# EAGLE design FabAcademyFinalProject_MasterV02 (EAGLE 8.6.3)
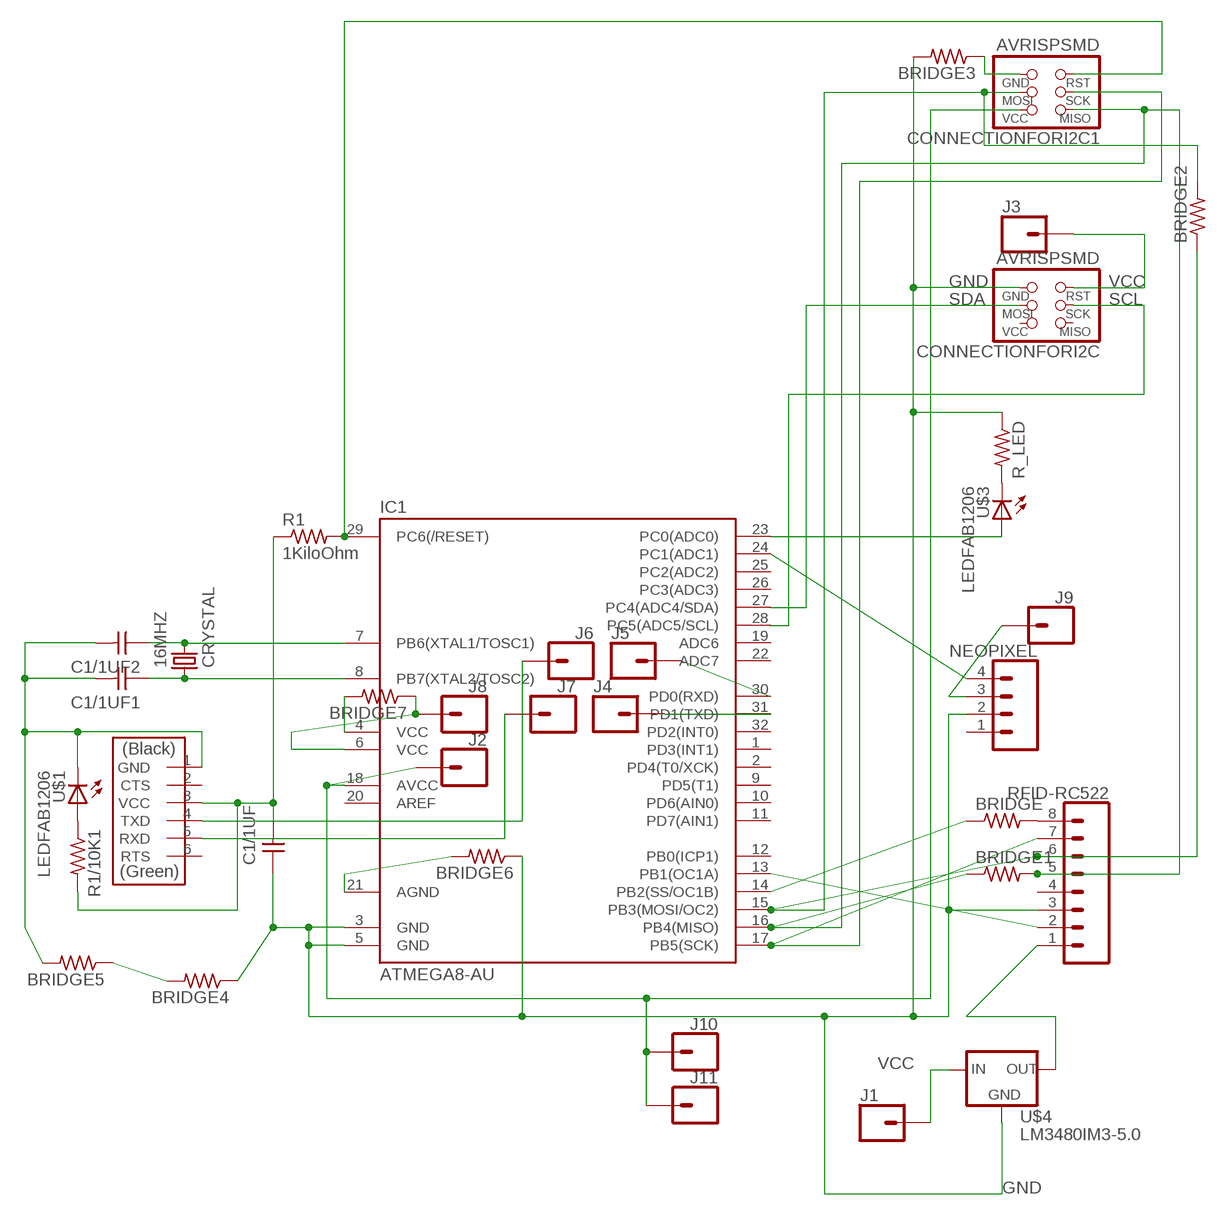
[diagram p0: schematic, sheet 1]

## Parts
16MHZ  CRYSTAL  [2-SMD-5X3MM]
BRIDGE  RES-US1206FAB  [R1206FAB]
BRIDGE1  RES-US1206FAB  [R1206FAB]
BRIDGE2  RES-US1206FAB  [R1206FAB]
BRIDGE3  RES-US1206FAB  [R1206FAB]
BRIDGE4  RES-US1206FAB  [R1206FAB]
BRIDGE5  RES-US1206FAB  [R1206FAB]
BRIDGE6  RES-US1206FAB  [R1206FAB]
BRIDGE7  RES-US1206FAB  [R1206FAB]
C1/1UF  CAP-UNPOLARIZEDFAB  [C1206FAB]
C1/1UF1  CAP-UNPOLARIZEDFAB  [C1206FAB]
C1/1UF2  CAP-UNPOLARIZEDFAB  [C1206FAB]
CONNECTIONFORI2C  AVRISPSMD  [2X03SMD]
CONNECTIONFORI2C1  AVRISPSMD  [2X03SMD]
IC1  ATMEGA8-AU  [TQFP32-08]
J1  CONN_01  [1X01]
J2  CONN_01  [1X01]
J3  CONN_01  [1X01]
J4  CONN_01  [1X01]
J5  CONN_01  [1X01]
J6  CONN_01  [1X01]
J7  CONN_01  [1X01]
J8  CONN_01  [1X01]
J9  CONN_01  [1X01]
J10  CONN_01  [1X01]
J11  CONN_01  [1X01]
NEOPIXEL  CONN_04  [1X04]
R1  1KiloOhm  RES-US1206FAB  [R1206FAB]
R1/10K1  RES-US1206FAB  [R1206FAB]
R_LED  RES-US1206FAB  [R1206FAB]
RFID-RC522  CONN_08"  [1X08]
U$1  LEDFAB1206  [LED1206FAB]
U$2  FTDI-SMD-HEADER  [1X06SMD]
U$3  LEDFAB1206  [LED1206FAB]
U$4  LM3480IM3-5.0  [SOT23]

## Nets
3.3V: RFID-RC522.1 U$4.1(OUT)
DI: IC1.24(PC1(ADC1)) NEOPIXEL.4
GND: BRIDGE3.2 BRIDGE4.1 BRIDGE5.2 BRIDGE6.1 C1/1UF1.2 C1/1UF2.2 C1/1UF.1 CONNECTIONFORI2C.6(GND) IC1.3(GND) IC1.5(GND) NEOPIXEL.2 R_LED.1 RFID-RC522.3 U$1.2(C) U$2.1(GND) U$4.3(GND)
N$1: IC1.13(PB1(OC1A)) RFID-RC522.2
N$2: CONNECTIONFORI2C1.3(SCK) IC1.17(PB5(SCK)) RFID-RC522.7
N$3: BRIDGE3.1 CONNECTIONFORI2C1.6(GND)
N$4: BRIDGE1.1 BRIDGE1.2 CONNECTIONFORI2C1.1(MISO) IC1.16(PB4(MISO)) RFID-RC522.5
N$5: BRIDGE.1 IC1.14(PB2(SS/OC1B))
N$6: 16MHZ.P$2 C1/1UF2.1 IC1.7(PB6(XTAL1/TOSC1))
N$7: 16MHZ.P$1 C1/1UF1.1 IC1.8(PB7(XTAL2/TOSC2))
N$8: J6.1 U$2.4(TXD)
N$9: R_LED.2 U$3.2(C)
N$10: IC1.23(PC0(ADC0)) U$3.1(A)
N$11: J7.1 U$2.5(RXD)
N$12: R1/10K1.1 U$1.1(A)
N$13: CONNECTIONFORI2C1.5(RST) IC1.29(PC6(/RESET)) R1.2
N$14: BRIDGE.2 RFID-RC522.8
N$15: BRIDGE2.1 BRIDGE2.2 CONNECTIONFORI2C1.4(MOSI) IC1.15(PB3(MOSI/OC2)) RFID-RC522.6
N$16: BRIDGE6.2 IC1.21(AGND)
N$17: BRIDGE4.2 BRIDGE5.1
N$18: IC1.30(PD0(RXD)) J5.1
N$19: IC1.31(PD1(TXD)) J4.1
N$20: BRIDGE7.2 IC1.4(VCC)
SCL: CONNECTIONFORI2C.3(SCK) IC1.28(PC5(ADC5/SCL))
SDA: CONNECTIONFORI2C.4(MOSI) IC1.27(PC4(ADC4/SDA))
VCC: BRIDGE7.1 C1/1UF.2 CONNECTIONFORI2C1.2(VCC) CONNECTIONFORI2C.5(RST) IC1.6(VCC) IC1.18(AVCC) J1.1 J2.1 J3.1 J8.1 J9.1 J10.1 J11.1 NEOPIXEL.3 R1.1 R1/10K1.2 U$2.3(VCC) U$4.2(IN)
Unconnected: CONNECTIONFORI2C.1(MISO) CONNECTIONFORI2C.2(VCC) IC1.1(PD3(INT1)) IC1.2(PD4(T0/XCK)) IC1.9(PD5(T1)) IC1.10(PD6(AIN0)) IC1.11(PD7(AIN1)) IC1.12(PB0(ICP1)) IC1.19(ADC6) IC1.20(AREF) IC1.22(ADC7) IC1.25(PC2(ADC2)) IC1.26(PC3(ADC3)) IC1.32(PD2(INT0)) NEOPIXEL.1 RFID-RC522.4 U$2.2(CTS) U$2.6(RTS)

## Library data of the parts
16MHZ = fab:CRYSTAL
BRIDGE BRIDGE1-BRIDGE7 R1 R1/10K1 R_LED = fab:RES-US: Resistor (US Symbol)
C1/1UF C1/1UF1 C1/1UF2 = fab:CAP-UNPOLARIZED
CONNECTIONFORI2C CONNECTIONFORI2C1 = fab:AVRISP
IC1 = atmega8:ATMEGA8
J1-J11 = SparkFun-Connectors:CONN_01: Single connection point. Often used as Generic Header-pin footprint for 0.1 inch spaced/style header connections
NEOPIXEL = SparkFun-Connectors:CONN_04: Multi connection point. Often used as Generic Header-pin footprint for 0.1 inch spaced/style header connections On any of the 0.1 inch spaced packages, you can populate with these: Break Away Headers - Straight (PRT-00116) Break Away Male Headers - Right Angle (PRT-00553) Female Headers (PRT-00115)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; PROD_ID: CONN-09696
RFID-RC522 = SparkFun-Connectors:CONN_08: Multi connection point. Often used as Generic Header-pin footprint for 0.1 inch spaced/style header connections On any of the 0.1 inch spaced packages, you can populate with these: Break Away Headers - Straight (PRT-00116) Break Away Male Headers - Right Angle (PRT-00553) Female Headers (PRT-00115)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; PROD_ID: CONN-08438
U$1 U$3 = fab:LED: LED
U$2 = fab:FTDI-SMD-HEADER
U$4 = national_gaui:LM3480

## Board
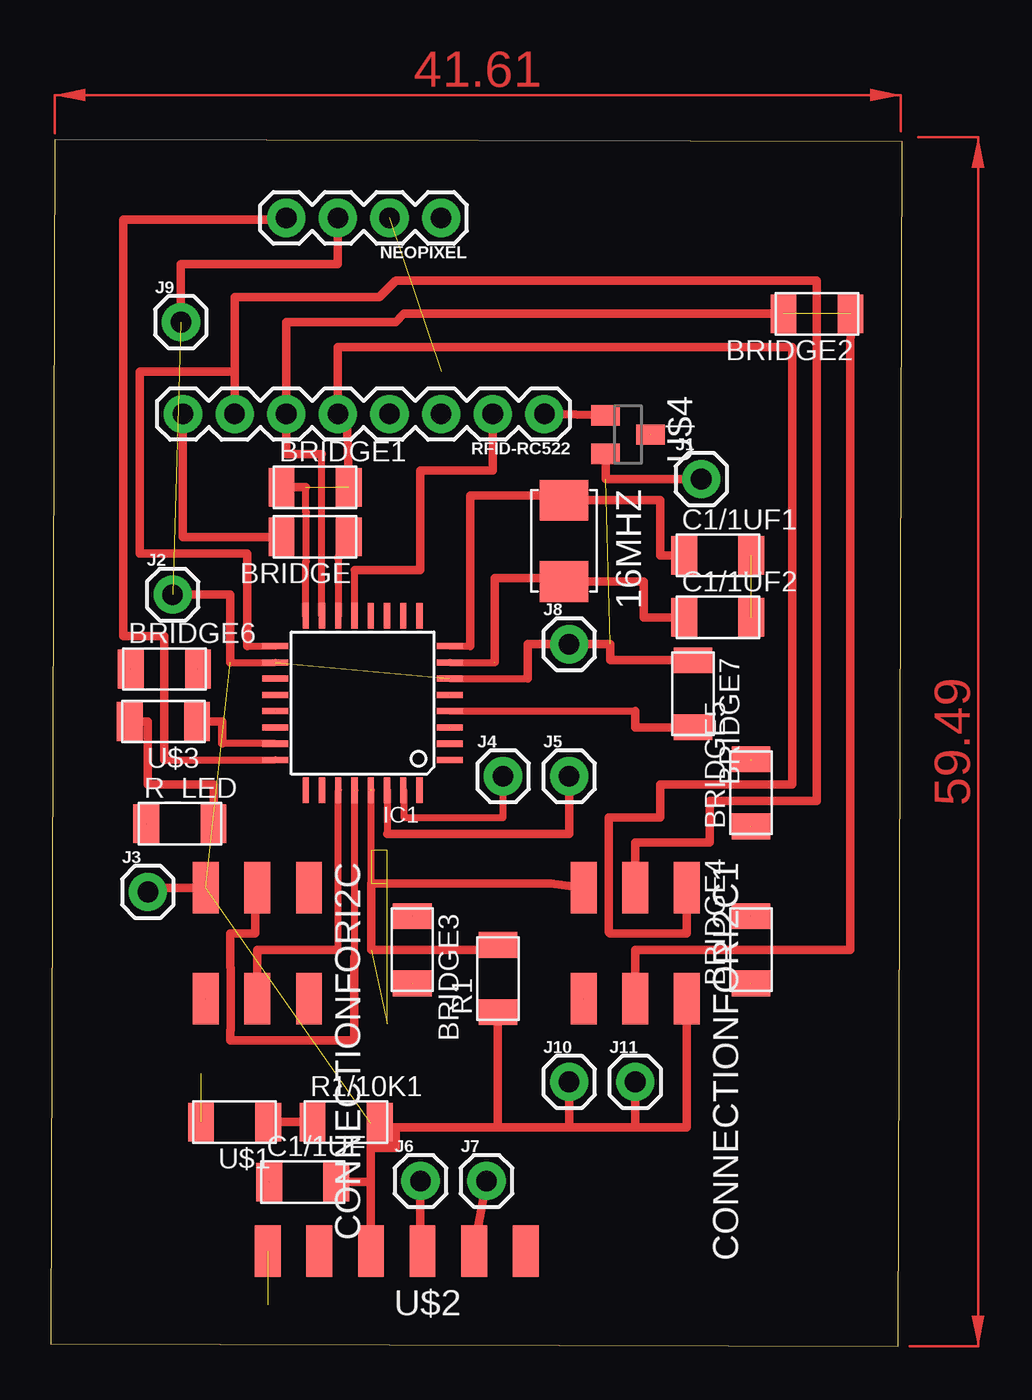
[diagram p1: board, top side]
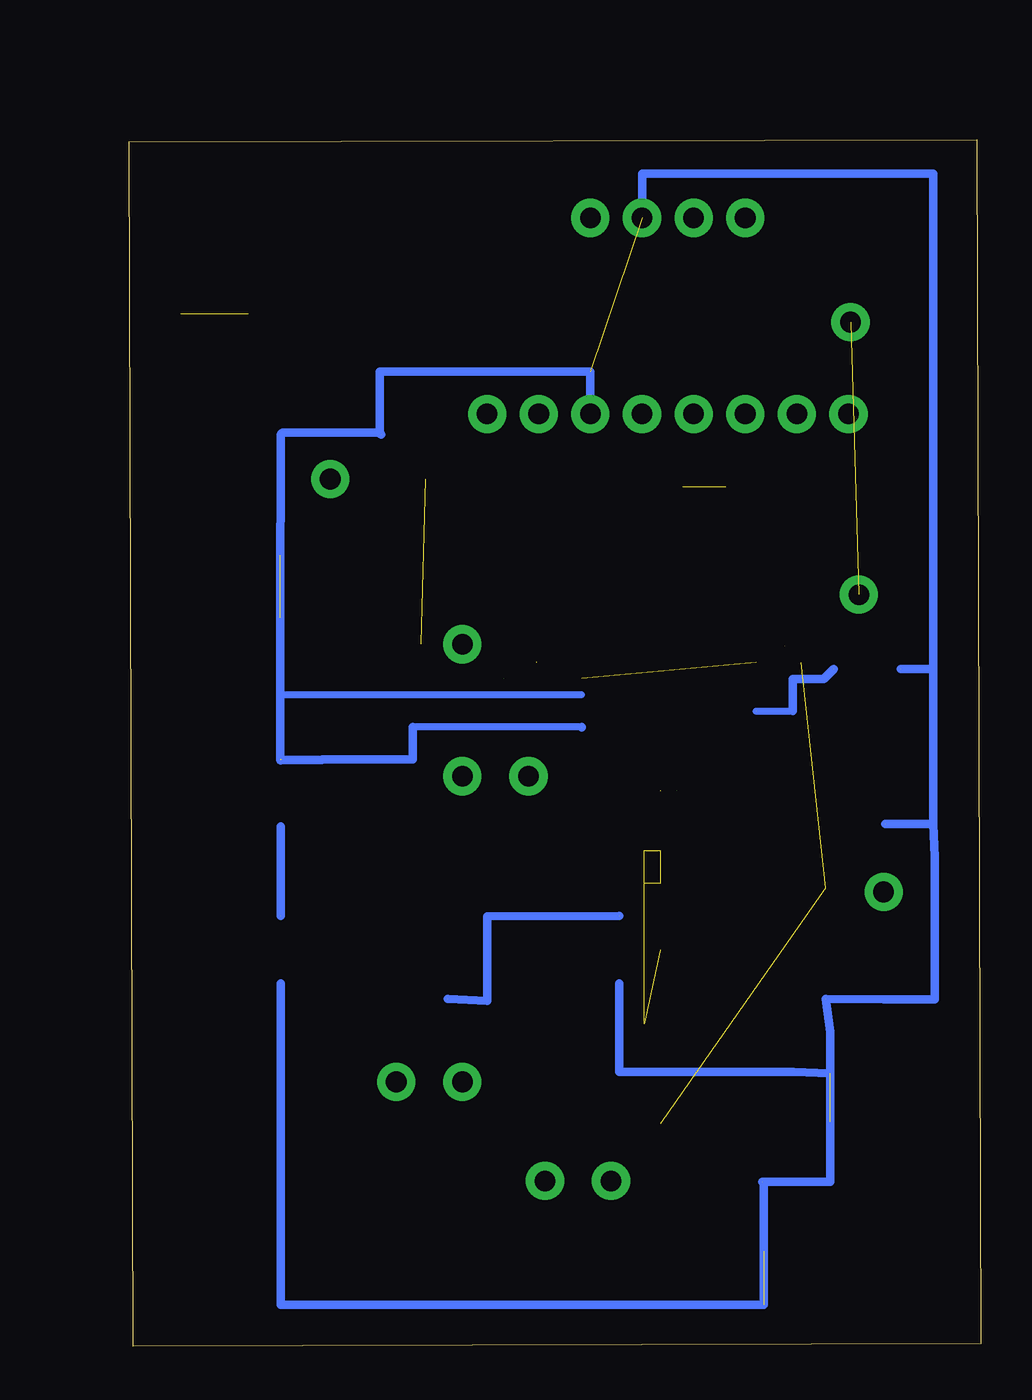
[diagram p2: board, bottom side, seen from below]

Size 41.88 x 59.38 mm. Coordinates in mm from the lower left corner, seen from the top.
Outline: 0,0.1 41.68,0 41.88,59.27 0.2,59.38 0,0.1
Copper layers (1*16): Top 0.035mm / dielectric 1.5mm / Bottom 0.035mm
Design rules "default *": minimum track width 6mil, minimum drill 0.35mm, track to track 16mil, track to pad 16mil, pad to pad 16mil, via to via 16mil, smd to smd 16mil, copper to edge 40mil, drill to drill 6mil, minimum pad ring 10mil, minimum via ring 8mil, stop-mask expansion 4mil, vias tented up to drill 0mil, thermal gap 10mil

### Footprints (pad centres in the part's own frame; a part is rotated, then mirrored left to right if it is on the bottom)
2-SMD-5X3MM = smd 2 x 2.4: P$1 -2,0; P$2 2,0
R1206FAB = smd 1.27 x 1.905: 1 -1.651,0; 2 1.651,0
C1206FAB = smd 1.27 x 1.905: 1 -1.651,0; 2 1.651,0
2X03SMD = smd 2.54 x 1.27: 1 -2.54,2.54; 2 2.92,2.54; 3 -2.54,0; 4 2.92,0; 5 -2.54,-2.54; 6 2.92,-2.54
TQFP32-08 = smd 1.27 x 0.305: 1 -4.293,2.8; 2 -4.293,2; 3 -4.293,1.2; 4 -4.293,0.4; 5 -4.293,-0.4; 6 -4.293,-1.2; 7 -4.293,-2; 8 -4.293,-2.8; 17 4.293,-2.8; 18 4.293,-2; 19 4.293,-1.2; 20 4.293,-0.4; 21 4.293,0.4; 22 4.293,1.2; 23 4.293,2; 24 4.293,2.8 | smd 0.305 x 1.27: 9 -2.8,-4.293; 10 -2,-4.293; 11 -1.2,-4.293; 12 -0.4,-4.293; 13 0.4,-4.293; 14 1.2,-4.293; 15 2,-4.293; 16 2.8,-4.293; 25 2.8,4.293; 26 2,4.293; 27 1.2,4.293; 28 0.4,4.293; 29 -0.4,4.293; 30 -1.2,4.293; 31 -2,4.293; 32 -2.8,4.293
1X01 = drill 1.016 pad 1.88: 1 0,0
1X04 = drill 1.016 pad 1.88: 1 0,0; 2 2.54,0; 3 5.08,0; 4 7.62,0
1X08 = drill 1.016 pad 1.88: 1 0,0; 2 2.54,0; 3 5.08,0; 4 7.62,0; 5 10.16,0; 6 12.7,0; 7 15.24,0; 8 17.78,0
LED1206FAB = smd 1.27 x 1.905: 1 -1.651,0; 2 1.651,0
1X06SMD = smd 2.54 x 1.27: 1 0,6.35; 2 0,3.81; 3 0,1.27; 4 0,-1.27; 5 0,-3.81; 6 0,-6.35
SOT23 = smd 1 x 1.4: 1 -0.95,-1.1; 2 0.95,-1.1; 3 0,1.1

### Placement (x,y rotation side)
16MHZ  25.25,39.62 270 top
BRIDGE  13,39.83 180 top
BRIDGE1  13,42.27 0 top
BRIDGE2  37.69,50.8 180 top
BRIDGE3  17.78,19.51 270 top
BRIDGE4  34.44,19.51 90 top
BRIDGE5  34.44,27.23 90 top
BRIDGE6  5.59,33.32 0 top
BRIDGE7  31.6,32.11 270 top
C1/1UF  12.4,8.08 0 top
C1/1UF1  32.82,38.91 0 top
C1/1UF2  32.82,35.86 0 top
CONNECTIONFORI2C  10.16,20.02 270 top
CONNECTIONFORI2C1  28.75,20.02 270 top
IC1  15.34,31.65 180 top
J1  32,42.67 0 top
J2  5.99,36.98 0 top
J3  4.78,22.35 0 top
J4  22.25,28.04 0 top
J5  25.5,28.04 0 top
J6  18.19,8.13 0 top
J7  21.44,8.13 0 top
J8  25.5,34.54 0 top
J9  6.4,50.39 0 top
J10  25.5,13 0 top
J11  28.75,13 0 top
NEOPIXEL  19.2,55.52 180 top
R1  22,18.08 90 top
R1/10K1  14.53,11.02 0 top
R_LED  6.35,25.7 0 top
RFID-RC522  24.28,45.87 180 top
U$1  9.04,11.02 180 top
U$2  17.02,4.67 90 top
U$3  5.54,30.73 180 top
U$4  28.4,44.86 270 top

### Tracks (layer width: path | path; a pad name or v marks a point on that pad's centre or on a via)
3.3V
  Top 0.406: RFID-RC522.1 24.45,45.87 U$4.1
DI
  Top 0.356: 5.59,28.85 IC1.24
  Top 0.406: NEOPIXEL.4 11.44,55.43 3.56,55.43 3.56,34.95 5.59,34.95 5.59,28.85
GND  (15 unrouted)
  Bottom 0.356: 19.63,30.48 27.94,30.48 | IC1.5 34.44,32.05
  Bottom 0.406: NEOPIXEL.2 16.66,57.71 2.34,57.71 2.34,33.32 | 7.39,13.41 7.39,15.47 CONNECTIONFORI2C.6 4.78,17.07 2.26,17.07 2.26,24.08 2.34,25.7 | 7.39,13.41 9.21,13.49 17.78,13.49 BRIDGE3.2 | RFID-RC522.3 19.2,47.96 29.57,47.96 29.57,44.92 U$4.3 29.66,44.96 34.34,44.96 34.44,44.86 34.44,42.16 C1/1UF1.2 34.47,32.05 | IC1.3 19.63,30.48 | 10.67,8.08 10.67,2.03 34.44,2.03 BRIDGE4.1 | 7.39,13.41 7.39,8.08 10.67,8.08 | 10.67,8.08 C1/1UF.1 | R_LED.1 2.34,25.7 | 2.34,33.32 BRIDGE6.1 | 2.34,25.7 2.34,33.32 | 27.94,30.48 27.94,28.88 32.39,28.88 32.42,28.85 34.47,28.85 | 34.44,32.05 34.47,32.05 | 34.47,28.85 34.45,28.83 | 34.47,32.05 34.47,28.85
N$1
  Top 0.356: IC1.13 14.94,38.2
  Top 0.406: RFID-RC522.2 21.74,43.08 18.19,43.08 18.19,38.2 14.94,38.2
N$2  (1 unrouted)
  Top 0.356: 9.65,34.45 IC1.17
  Top 0.406: RFID-RC522.7 9.04,47.96 | 9.04,47.96 4.37,47.96 4.37,39.01 9.65,39.01 9.65,34.46 | 9.04,47.96 9.04,51.61 16.15,51.61 16.97,52.43 37.69,52.43 37.69,26.82 32.41,26.82 32.41,24.79 28.75,24.79 CONNECTIONFORI2C1.3
N$3  (2 unrouted)
  Bottom 0.406: CONNECTIONFORI2C1.6 24.28,16.99 24.28,21.13 BRIDGE3.1
N$4  (1 unrouted)
  Top 0.356: IC1.16 12.54,38.6 12.57,38.63 12.57,41.02 12.54,41.05 12.54,42.27
  Top 0.406: 12.54,42.27 BRIDGE1.1 | CONNECTIONFORI2C1.1 31.29,20.32 27.51,20.32 27.46,20.37 27.46,26.01 29.97,26.01 29.97,27.64 36.47,27.64 36.47,49.17 14.12,49.17 RFID-RC522.5 14.55,45.87 BRIDGE1.2
N$5
  Top 0.356: 14.15,38.79 IC1.14
  Top 0.406: BRIDGE.1 14.15,38.79
N$6  (1 unrouted)
  Top 0.356: IC1.7 21.84,33.65
  Top 0.406: C1/1UF2.1 29.16,35.86 29.16,37.62 16MHZ.P$2 25.25,37.8 21.84,37.8 21.84,33.66
N$7
  Top 0.356: IC1.8 20.62,34.45
  Top 0.406: 20.62,34.45 20.62,41.86 25.25,41.86 16MHZ.P$1 29.97,41.62 29.97,38.91 C1/1UF1.1
N$8
  Top 0.406: U$2.4 18.29,4.88 18.19,4.47 J6.1
N$9
  Top 0.406: 4.72,30.73 U$3.2 4.78,30.73 4.78,27.64 6.46,27.64 6.47,27.63 8.03,27.63 8.03,26.11 R_LED.2
N$10
  Top 0.356: IC1.23 8.43,29.65
  Top 0.406: U$3.1 8.43,30.73 8.43,29.65
N$11
  Top 0.406: U$2.5 20.83,4.88 J7.1
N$12
  Top 0.406: R1/10K1.1 U$1.1
N$13  (7 unrouted)
  Top 0.356: 15.77,22.76 15.77,27.36
  Top 0.406: R1.2 21.77,19.91 21.84,19.51 15.77,19.51 15.77,22.76 24.59,22.76 CONNECTIONFORI2C1.5
N$14
  Top 0.406: RFID-RC522.8 6.5,39.83 BRIDGE.2
N$15  (1 unrouted)
  Top 0.356: IC1.15 13.34,43.89
  Top 0.406: 13.34,43.89 11.58,43.89 RFID-RC522.6 11.58,50.39 16.97,50.39 17.37,50.8 BRIDGE2.2 | CONNECTIONFORI2C1.4 28.75,19.51 39.32,19.51 39.32,48.36 BRIDGE2.1
N$16  (2 unrouted)
  Bottom 0.356: IC1.21 9.25,31.25
  Bottom 0.406: BRIDGE6.2 7.73,32.84 9.25,32.84 9.25,31.25
N$17  (2 unrouted)
  Bottom 0.406: BRIDGE4.2 BRIDGE5.1
N$18
  Top 0.356: IC1.30 16.56,27.36 16.56,25.2
  Top 0.406: 16.56,25.2 25.5,25.2 J5.1
N$19
  Top 0.356: IC1.31 17.37,27.32 17.37,26.01 22.25,26.01 J4.1
N$20
  Top 0.356: IC1.4 28.75,31.25
  Top 0.406: BRIDGE7.2 28.75,30.45 28.75,31.24 | 28.75,31.24 | 28.75,31.25 28.75,31.24
SCL  (1 unrouted)
  Top 0.356: 14.95,19.17 14.95,27.36
  Top 0.406: CONNECTIONFORI2C.3 10.06,22.56 10.06,20.32 8.84,20.32 8.84,18.64 8.86,18.62 8.86,15.57 8.84,15.55 8.84,15.04 14.94,15.04 14.94,19.15 14.95,19.17
SDA
  Top 0.356: 14.14,19.51 IC1.27
  Top 0.406: CONNECTIONFORI2C.4 10.16,19.51 14.14,19.51
VCC  (6 unrouted)
  Top 0.356: 8.84,33.65 IC1.18 | IC1.6 23.47,32.85
  Top 0.406: CONNECTIONFORI2C1.2 31.29,10.77 28.75,10.77 | U$4.2 27.3,42.67 J1.1 | J2.1 8.84,36.98 8.84,33.65 | CONNECTIONFORI2C.5 4.78,22.56 J3.1 | BRIDGE7.1 27.53,33.76 27.53,34.54 J8.1 23.47,34.54 23.47,32.86 | 25.5,10.77 28.75,10.77 | J9.1 6.4,53.24 14.12,53.24 NEOPIXEL.3 | J10.1 25.5,10.77 | J11.1 28.75,10.77 | R1.1 22,10.77 | 22,10.77 25.5,10.77 | 16.97,10.77 16.18,10.77 R1/10K1.2 16.15,11.02 16.15,10.97 15.75,10.97 15.75,10.16 | 16.97,10.77 22,10.77 | C1/1UF.2 15.75,8.08 U$2.3 15.75,9.75 | 15.75,9.75 15.75,10.16 | 15.75,9.75 16.97,9.75 16.97,10.16 | 16.97,10.77 16.97,10.16 | 15.75,10.16 16.97,10.16
(copper drawn outside any net)
  shapes: Top area x2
